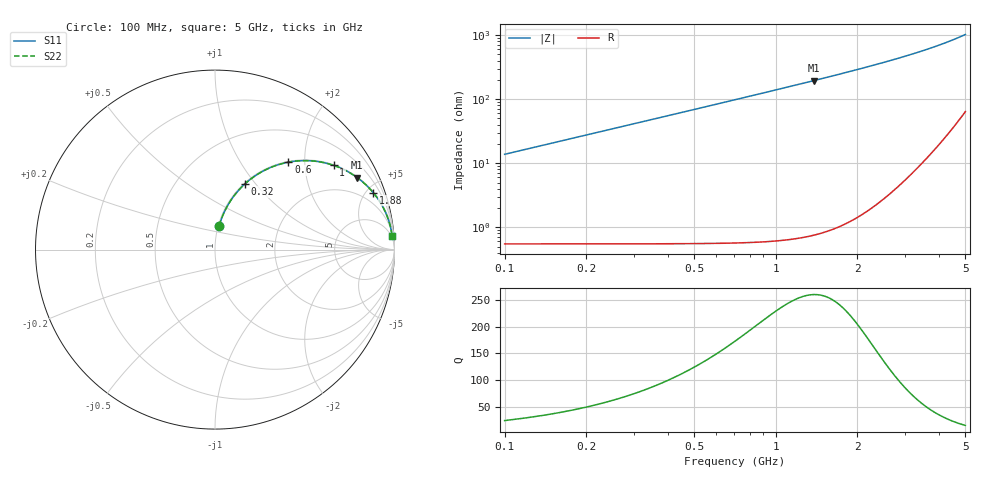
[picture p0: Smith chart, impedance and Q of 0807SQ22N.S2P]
! Coilcraft 0807SQ-22N Air Core Inductor
! 07 March 2008
# MHZ S MA R 50
!Freq  MagS11  AngS11  MagS21  AngS21  MagS12  AngS12  MagS22  AngS22
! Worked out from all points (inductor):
!   246 points, 100 MHz to 5 GHz, reference 50 ohm
!   read as one part in series: L = 21.9 nH near 120 MHz
!   highest Q = 259 at 1.38 GHz (marker M1), where L = 22.5 nH
!   S11 on the Smith chart (normalised r, x): 100 MHz: 1.01, +0.28; 320 MHz: 1.01, +0.88; 600 MHz: 1.01, +1.66; 1 GHz: 1.02, +2.80; 1.88 GHz: 1.07, +5.53; 5 GHz: 4, +25
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100  0.1356 79.9  0.9854 -7.8  0.9854 -7.8  0.1356 79.9
120  0.1621 78.7  0.9814 -9.3  0.9814 -9.3  0.1621 78.7
140  0.1882 77.5  0.9768 -10.9  0.9768 -10.9  0.1882 77.5
160  0.2139 76.2  0.9715 -12.4  0.9715 -12.4  0.2139 76.2
200  0.264 73.5  0.9593 -15.3  0.9593 -15.3  0.264 73.5
260  0.3353 69.5  0.937 -19.6  0.937 -19.6  0.3353 69.5
320  0.4014 65.6  0.9109 -23.7  0.9109 -23.7  0.4014 65.6
380  0.4619 61.8  0.8821 -27.6  0.8821 -27.6  0.4619 61.8
440  0.5166 58.3  0.8515 -31.2  0.8515 -31.2  0.5166 58.3
520  0.5809 53.9  0.8094 -35.6  0.8094 -35.6  0.581 53.9
600  0.6362 50.0  0.7673 -39.6  0.7673 -39.6  0.6362 50.0
760  0.7233 43.2  0.6867 -46.5  0.6867 -46.5  0.7233 43.2
920  0.7862 37.7  0.6143 -52.0  0.6143 -52.0  0.7862 37.7
1000  0.8108 35.4  0.5817 -54.4  0.5817 -54.4  0.8109 35.4
1180  0.8542 30.8  0.5166 -58.9  0.5166 -58.9  0.8542 30.8
1380  0.8882 26.8  0.4561 -62.9  0.4561 -62.9  0.8882 26.8
1740  0.9268 21.4  0.3716 -68.3  0.3716 -68.3  0.9268 21.4
1880  0.9369 19.8  0.3452 -69.9  0.3452 -69.9  0.937 19.8
2560  0.9662 14.0  0.2504 -75.6  0.2504 -75.6  0.9662 14.0
3380  0.9809 9.6  0.1789 -79.5  0.1789 -79.5  0.9809 9.6
4200  0.987 6.6  0.1309 -81.5  0.1309 -81.5  0.9871 6.6
5000  0.9893 4.4  0.09654 -82.0  0.09654 -82.0  0.9893 4.4
